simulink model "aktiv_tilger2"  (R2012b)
settings: Solver=ode45  StartTime=0.0  StopTime=10.0  RelTol=1e-3
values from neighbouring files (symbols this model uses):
  a11 = a11{:}    [aktiv_tilger_2.m]    (also in aktiv_tilger_3.m; aktiv_tilger_31.m)
  a12 = a12{:}    [aktiv_tilger_2.m]    (also in aktiv_tilger_3.m; aktiv_tilger_31.m)
  a21 = a21{:}    [aktiv_tilger_2.m]    (also in aktiv_tilger_3.m; aktiv_tilger_31.m)
  a22 = a22{:}    [aktiv_tilger_2.m]    (also in aktiv_tilger_3.m; aktiv_tilger_31.m)
  b11 = b11{:}    [aktiv_tilger_2.m]    (also in aktiv_tilger_3.m; aktiv_tilger_31.m)
  b12 = b12{:}    [aktiv_tilger_2.m]    (also in aktiv_tilger_3.m; aktiv_tilger_31.m)
  b21 = b21{:}    [aktiv_tilger_2.m]    (also in aktiv_tilger_3.m; aktiv_tilger_31.m)
  b22 = b22{:}    [aktiv_tilger_2.m]    (also in aktiv_tilger_3.m; aktiv_tilger_31.m)
  fsig = 0.01    [aktiv_tilger_1.m]    (also in aktiv_tilger_12.m = 0.1; aktiv_tilger_2.m = 2; aktiv_tilger_3.m = 0.1; diff_filter_1.m = 1)
  Kr = 2000    [aktiv_tilger_2.m]    (also in beobachter_22.m = 5; fuellstnd_3.m = 10,; fuellstnd_31.m = 10,; kalman_12.m = Kn(1:2))

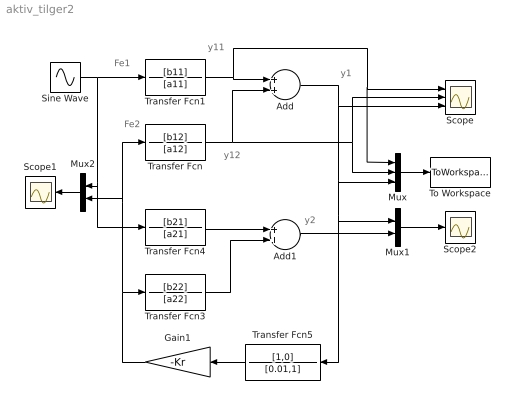
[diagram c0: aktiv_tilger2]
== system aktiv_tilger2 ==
  note: y2
  note: Fe2
  note: Fe1
  note: y1
  note: y12
  note: y11
  Add : Sum
  Add1 : Sum
  Gain1 : Gain  Gain=-Kr
  Mux : Mux  Inputs=3
  Mux1 : Mux  Inputs=2
  Mux2 : Mux  Inputs=2
  Scope : Scope  NumInputPorts=3
  Scope1 : Scope
  Scope2 : Scope
  Sine Wave : Sin  Amplitude=0.5  Frequency=fsig  SampleTime=0
  To Workspace : ToWorkspace  VariableName=y  SampleTime=-1  SaveFormat=Structure With Time
  Transfer Fcn : TransferFcn  Numerator=[b12]  Denominator=[a12]
  Transfer Fcn1 : TransferFcn  Numerator=[b11]  Denominator=[a11]
  Transfer Fcn3 : TransferFcn  Numerator=[b22]  Denominator=[a22]
  Transfer Fcn4 : TransferFcn  Numerator=[b21]  Denominator=[a21]
  Transfer Fcn5 : TransferFcn  Numerator=[1,0]  Denominator=[0.01,1]
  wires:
  Sine Wave/1 -> Mux2/1, Transfer Fcn4/1, Transfer Fcn1/1
  Mux/1 -> To Workspace/1
  Gain1/1 -> Mux2/2, Transfer Fcn/1, Transfer Fcn3/1
  Transfer Fcn/1 -> Scope/2, Mux/2, Add/2
  Transfer Fcn1/1 -> Mux/1, Scope/1, Add/1
  Transfer Fcn4/1 -> Add1/1
  Transfer Fcn3/1 -> Add1/2
  Add1/1 -> Mux1/2
  Mux1/1 -> Scope2/1
  Add/1 -> Scope/3, Transfer Fcn5/1, Mux1/1, Mux/3
  Transfer Fcn5/1 -> Gain1/1
  Mux2/1 -> Scope1/1
